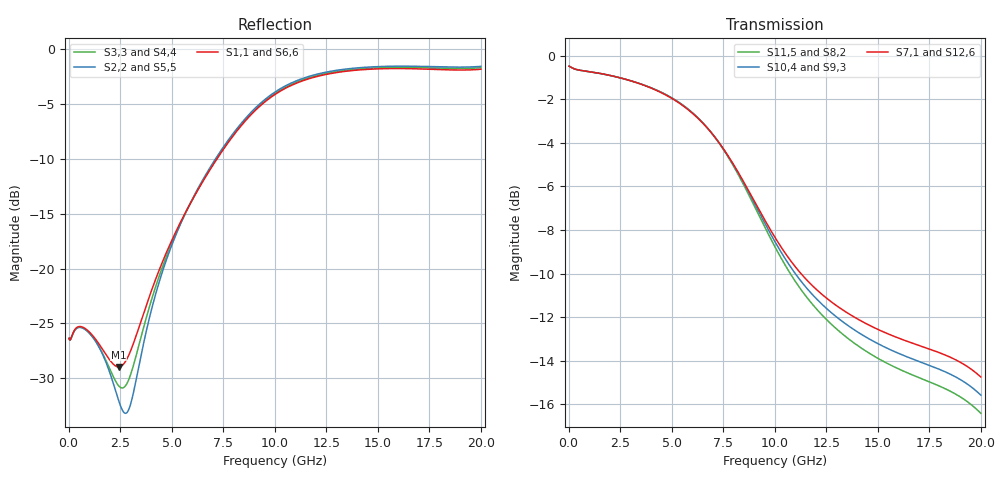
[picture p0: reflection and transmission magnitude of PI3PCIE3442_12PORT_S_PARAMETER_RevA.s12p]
! NPort=12 DATA=800 NOISE=0 GROUPDELAY=0 COMPLEX_DATAFORMAT=POLAR
! NumOfBlock=1 NumOfParam=0
! .MODEL Smodel S TSTONEFILE=PI3PCIE3442_12PORT_S_PARAMETER_RevA.s12p TYPE=S
!  -- The above .MODEL line can be used for the S element in the netlist.
! PORT DEFINITION
! PORT1 = INPUT1+
! PORT2 = INPUT1-
! PORT3 = INPUT2+
! PORT4 = INPUT2-
! PORT5 = INPUT3+
! PORT6 = INPUT3-
! PORT7 = OUTPUT1+
! PORT8 = OUTPUT1-
! PORT9  = OUTPUT2+
! PORT10 = OUTPUT2-
! PORT11 = OUTPUT3+
! PORT12 = OUTPUT3-
# Hz S MA R  50
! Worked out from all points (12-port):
!   800 points, 25 MHz to 20 GHz, reference 50 ohm
!   strongest paths, dB at 25 MHz, 5.025 GHz, 10.03 GHz, 15.03 GHz, 20 GHz:
!     S7,1: -0.5, -2.0, -8.4, -12.6, -14.8
!     S12,6: -0.5, -2.0, -8.4, -12.6, -14.8
!     S10,4: -0.5, -1.9, -8.6, -13.2, -15.6
!     S9,3: -0.5, -1.9, -8.6, -13.2, -15.6
!     S11,5: -0.5, -1.9, -8.8, -13.9, -16.4
!     S8,2: -0.5, -1.9, -8.8, -13.9, -16.4
!   lowest |S11| = -29.0 dB at 2.425 GHz (marker M1), VSWR 1.07, Z = 53.6 + j0.727 ohm
!   |S11| at or under -10 dB: start of sweep to 7.194 GHz
